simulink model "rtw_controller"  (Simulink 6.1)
settings: Solver=ode1  SolverMode=SingleTasking  StartTime=0.0  StopTime=.25  RelTol=1e-3  AbsTol=1e-6
undefined symbols (not defined in the file or in its folder): c_damping, k_stiffness

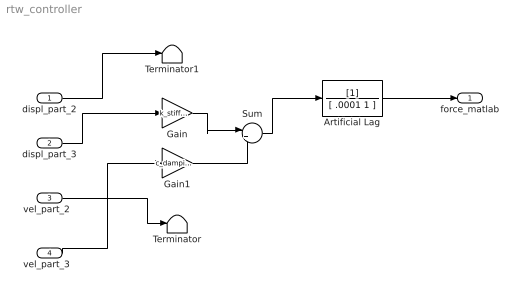
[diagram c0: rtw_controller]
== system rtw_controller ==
  displ_part_2 : Inport  Port=1  LatchInput=off
  displ_part_3 : Inport  Port=2  LatchInput=off
  "vel_part_2  " : Inport  Port=3  LatchInput=off
  "vel_part_3  " : Inport  Port=4  LatchInput=off
  Artificial Lag : TransferFcn  Denominator=[ .0001 1 ]
  Gain : Gain  Gain=k_stiffness
  Gain1 : Gain  Gain=c_damping
  Sum : Sum  Inputs=|++
  Terminator : Terminator
  Terminator1 : Terminator
  force_matlab : Outport
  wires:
  Gain/1 -> Sum/1
  Gain1/1 -> Sum/2
  displ_part_3/1 -> Gain/1
  "vel_part_3  "/1 -> Gain1/1
  Artificial Lag/1 -> force_matlab/1
  Sum/1 -> Artificial Lag/1
  "vel_part_2  "/1 -> Terminator/1
  displ_part_2/1 -> Terminator1/1
